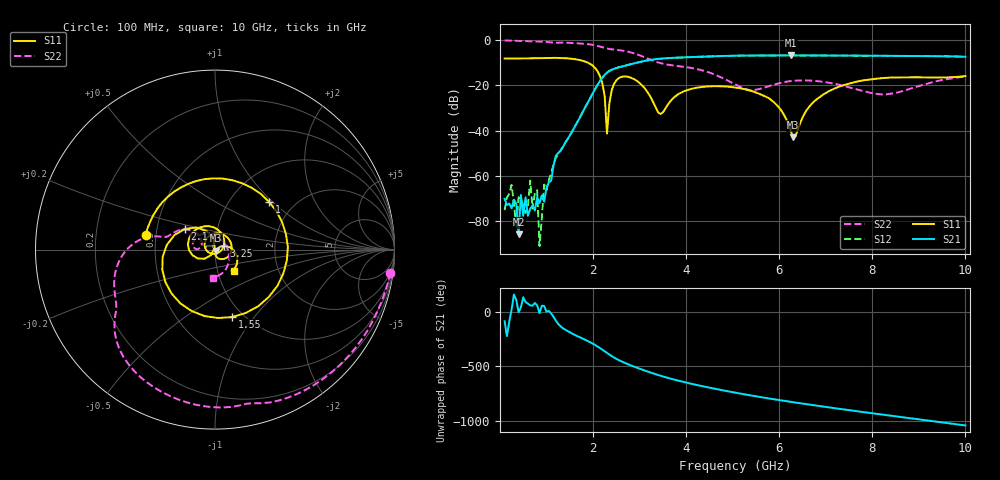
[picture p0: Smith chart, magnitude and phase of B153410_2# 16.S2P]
!  2-Port S-parameters saved by WinCal
! VAR MeasName=S-Parameters (CALIBRATED_DATA) read from VNA (N5245A)
! VAR MeasDate=2016-12-23 10:00:08
! VAR NAME=B153410_2# 16
! VAR FILENAME=B153410_2# 16.S2P
! VAR DATE=2016-12-23 10:00:08
! VAR PHYS_PORTS=1,2
# Hz S DB R 50
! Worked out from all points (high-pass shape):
!   199 points, 100 MHz to 10 GHz, reference 50 ohm
!   highest |S21| = -6.73 dB at 6.25 GHz (marker M1); lowest = -85.7 dB at 400 MHz (marker M2)
!   |S21| within 3 dB of the highest: 2.984 GHz to end of sweep
!   lowest |S11| = -42.8 dB at 6.3 GHz (marker M3), VSWR 1.01, Z = 50.5 - j0.532 ohm
!   |S11| at or under -10 dB: 1.894 GHz to end of sweep
!   |S22| runs from -24.0 to -0.1 dB; largest |S21 - S12| = 0.0031
!   S11 on the Smith chart (normalised r, x): 100 MHz: 0.44, +0.08; 1 GHz: 1.50, +0.95; 1.55 GHz: 0.89, -0.78; 2.1 GHz: 0.70, +0.17; 3.25 GHz: 1.10, +0.04; 10 GHz: 1.20, -0.30
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1e8  -8.08 168.3  -70.05 -83.9  -75.05 -32.3  -0.13 -7.5
2.5e8  -8.10 150.6  -74.31 22.9  -63.89 102.0  -0.24 -17.6
3.5e8  -8.07 138.3  -72.22 113.9  -82.48 31.9  -0.31 -24.3
4e8  -8.08 132.2  -85.72 -1.0  -69.41 -125.3  -0.33 -27.6
5.5e8  -8.06 112.4  -69.43 93.2  -76.31 34.4  -0.42 -37.5
6.5e8  -8.03 98.5  -74.47 62.6  -62.07 11.1  -0.48 -44.1
8.5e8  -7.97 67.7  -72.04 -9.0  -91.00 113.8  -0.63 -57.2
1e9  -7.91 41.6  -65.19 4.2  -66.39 28.4  -0.79 -67.0
1.55e9  -8.23 -75.6  -40.37 162.4  -40.45 162.5  -1.25 -100.4
1.75e9  -8.96 -122.5  -32.85 122.2  -32.80 121.8  -1.51 -113.5
2.1e9  -13.86 145.2  -19.63 42.7  -19.63 42.7  -2.55 -137.6
2.25e9  -24.66 98.0  -15.33 -1.6  -15.34 -1.5  -3.43 -145.8
2.3e9  -41.30 106.9  -14.36 -16.9  -14.36 -16.7  -3.70 -147.7
2.55e9  -16.80 -178.7  -12.01 -81.7  -12.01 -81.6  -4.39 -158.4
3.25e9  -25.61 22.0  -8.65 160.7  -8.66 160.8  -8.73 168.6
3.4e9  -31.98 -43.1  -8.29 139.9  -8.28 139.9  -9.85 166.8
5.05e9  -20.90 -7.1  -6.86 -22.4  -6.87 -22.2  -19.49 140.7
6.25e9  -40.19 -69.5  -6.73 -107.6  -6.75 -107.6  -18.04 169.9
6.3e9  -42.82 -46.8  -6.76 -111.0  -6.76 -110.9  -17.96 168.3
6.7e9  -28.11 27.6  -6.75 -136.1  -6.77 -136.1  -17.87 151.4
8.35e9  -16.57 -36.6  -6.93 127.4  -6.90 127.6  -23.77 25.7
1e10  -15.84 -48.5  -7.33 34.8  -7.32 35.1  -16.13 -94.8
